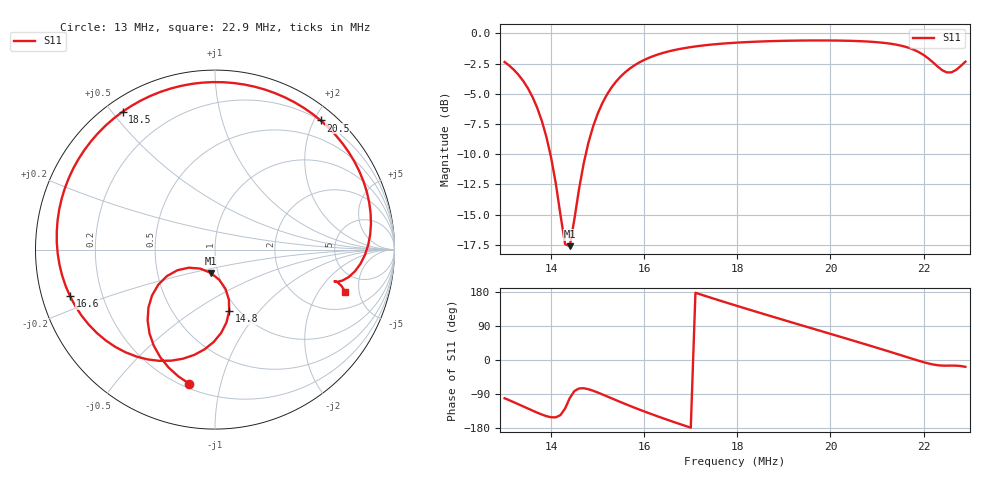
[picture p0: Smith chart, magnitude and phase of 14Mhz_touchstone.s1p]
# MHz Z RI R 50.0
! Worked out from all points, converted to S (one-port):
!   100 points, 13 MHz to 22.9 MHz, reference 50 ohm
!   lowest |S11| = -17.6 dB at 14.4 MHz (marker M1), VSWR 1.30, Z = 46.1 - j12.1 ohm
!   |S11| at or under -10 dB: 13.98 MHz to 14.74 MHz (762 kHz wide, 5.31 % of centre)
!   S11 on the Smith chart (normalised r, x): 13 MHz: 0.23, -0.80; 14.8 MHz: 0.91, -0.71; 16.6 MHz: 0.08, -0.16; 18.5 MHz: 0.05, +0.53; 20.5 MHz: 0.20, +2.09; 22.9 MHz: 3.19, -3.61
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13  0.2257 -0.8001
13.4  0.2861 -0.5139
13.7  0.382 -0.326
14  0.5568 -0.181
14.3  0.8304 -0.179
14.4  0.9223 -0.243
14.6  1.015 -0.4704
14.8  0.9061 -0.7107
15  0.6832 -0.8085
15.2  0.4821 -0.7782
15.5  0.2896 -0.6418
15.7  0.2147 -0.5411
16  0.1465 -0.3996
16.6  0.0841 -0.1562
16.8  0.0735 -0.0831
17.4  0.0556 0.1264
18  0.0494 0.3383
18.5  0.0502 0.5322
19.2  0.0614 0.8653
19.8  0.0892 1.27
20.5  0.1972 2.094
21.1  0.7131 3.817
21.4  2.153 5.893
21.7  9.684 6.61
22.1  5.926 -3.822
22.5  3.663 -2.479
22.7  3.741 -2.703
22.9  3.192 -3.609
